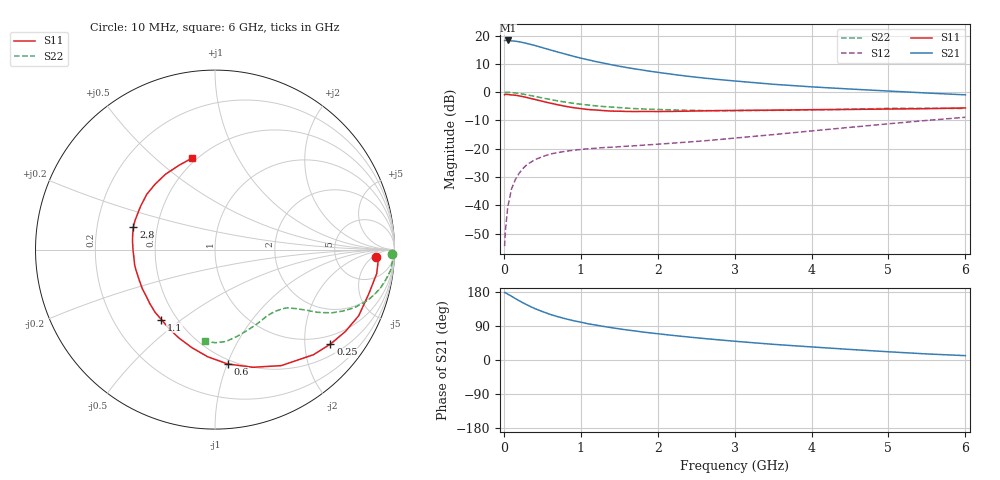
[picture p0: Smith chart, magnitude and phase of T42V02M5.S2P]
! Infineon Technologies  Discrete & RF Semiconductors
! BFR182T
! Si NPN RF Bipolar Junction Transistor in SC75
! VCE = 2 V  IC = 2.5 mA
! Common Emitter S-Parameters:  October  1999
# GHz  S  MA  R  50
!  f  S11  S21  S12  S22
! GHz  MAG  ANG  MAG  ANG  MAG  ANG  MAG  ANG
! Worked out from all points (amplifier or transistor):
!   36 points, 10 MHz to 6 GHz, reference 50 ohm
!   highest |S21| = 18.3 dB at 50 MHz (marker M1)
!   |S21| within 3 dB of that: start of sweep to 560.1 MHz
!   unconditionally stable (mu >= 1): 1.814 GHz to 4.287 GHz
!   at 250 MHz: K = 0.17, MSG = 22.2 dB, |S12| = -27.0 dB
!   at 1.4 GHz: K = 0.85, MSG = 14.6 dB, |S12| = -19.5 dB
!   at 6 GHz: K = 0.84, MSG = 4.0 dB, |S12| = -8.9 dB
!   lowest NFmin = 1.10 dB at 450 MHz
!   S11 on the Smith chart (normalised r, x): 10 MHz: 15, -7; 250 MHz: 0.76, -2.60; 600 MHz: 0.46, -1.00; 1.1 GHz: 0.41, -0.42; 2.8 GHz: 0.36, +0.12; 6 GHz: 0.47, +0.66
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0.01  0.8985 -2.8  8.137 178.2  0.0019 80.2  0.988 -1.4
0.02  0.9129 -2.1  8.174 177.8  0.0035 86.4  0.9916 -1.3
0.05  0.911 -8.4  8.177 173.9  0.0092 87.7  0.9914 -3.5
0.1  0.8919 -15.9  8.045 168.2  0.0195 82.7  0.9844 -6.9
0.15  0.8814 -24.7  7.931 162.0  0.0286 76.7  0.9651 -10.1
0.25  0.8311 -39.3  7.502 150.8  0.0449 69.2  0.9212 -15.9
0.3  0.8023 -46.9  7.23 145.6  0.0524 66.0  0.8966 -18.4
0.4  0.7442 -60.3  6.688 135.9  0.0637 59.4  0.8404 -22.7
0.5  0.6887 -72.2  6.112 127.9  0.0724 55.0  0.7893 -25.7
0.6  0.641 -83.7  5.584 120.5  0.0804 51.1  0.7422 -28.3
0.7  0.5984 -93.9  5.111 114.4  0.0854 48.8  0.7001 -30.1
0.8  0.5619 -103.1  4.695 108.9  0.0901 46.4  0.6657 -31.6
0.9  0.5323 -112.1  4.312 104.0  0.0939 45.2  0.6346 -32.7
1.1  0.4915 -127.4  3.711 95.4  0.1001 43.6  0.5906 -34.5
1.3  0.4713 -140.5  3.249 88.5  0.1049 43.0  0.556 -36.2
1.6  0.4554 -157.2  2.711 79.3  0.111 43.7  0.5213 -38.5
2.2  0.4567 -179.7  2.055 64.8  0.1257 48.3  0.4851 -44.5
2.8  0.4718 164.4  1.666 53.1  0.1454 52.8  0.4691 -52.0
3.5  0.4798 149.8  1.377 41.4  0.1774 56.9  0.4768 -61.4
4.5  0.4942 132.6  1.134 27.9  0.2386 58.3  0.4993 -75.9
5.5  0.5105 113.3  0.964 16.0  0.3164 55.3  0.5188 -89.8
6  0.5253 104.2  0.895 11.5  0.3594 52.1  0.5139 -96.1
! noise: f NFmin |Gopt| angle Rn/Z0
0.45  1.1  0.39  29  0.35
0.9  1.2  0.37  59  0.28
1.8  1.8  0.28  128  0.2
